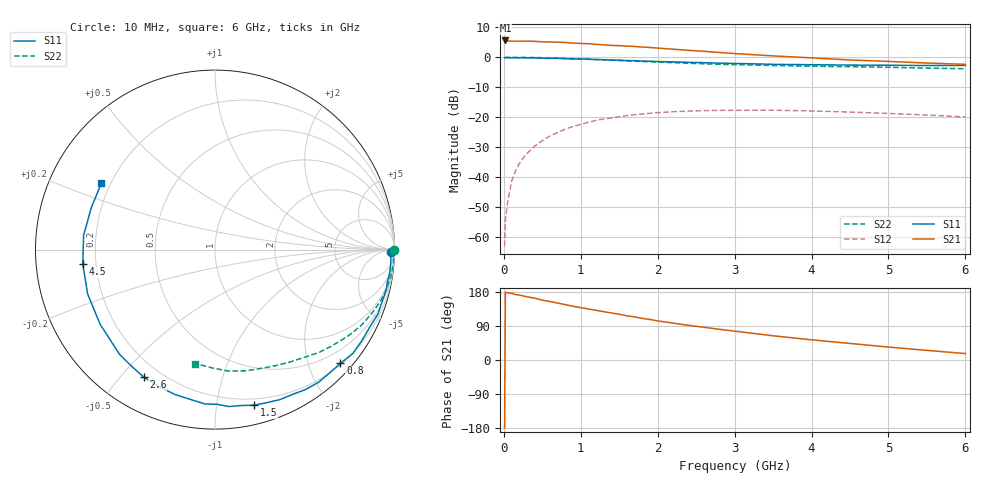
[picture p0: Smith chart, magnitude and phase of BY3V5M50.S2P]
! SIEMENS Small Signal Semiconductors
! BFY420
! Si NPN RF SIEGET Grounded Emitter Transistor in MICRO-X
! VCE = 3.5 V  IC = 0.5 mA
! Common Emitter S-Parameters:  October  1996
# GHz  S  MA  R  50
!  f  S11  S21  S12  S22
! GHz  MAG  ANG  MAG  ANG  MAG  ANG  MAG  ANG
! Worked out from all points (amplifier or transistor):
!   36 points, 10 MHz to 6 GHz, reference 50 ohm
!   highest |S21| = 5.6 dB at 20 MHz (marker M1)
!   |S21| within 3 dB of that: start of sweep to 2.243 GHz
!   unconditionally stable (mu >= 1): 4.7 GHz to end of sweep
!   at 250 MHz: K = 0.04, MSG = 19.5 dB, |S12| = -33.7 dB
!   at 1.4 GHz: K = 0.16, MSG = 12.1 dB, |S12| = -20.3 dB
!   at 6 GHz: K = 1.45, MAG = 4.8 dB, |S12| = -19.9 dB
!   S11 on the Smith chart (normalised r, x): 10 MHz: 76, -51; 800 MHz: 0.22, -2.57; 1.5 GHz: 0.15, -1.27; 2.6 GHz: 0.14, -0.58; 4.5 GHz: 0.15, -0.05; 6 GHz: 0.17, +0.26
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0.01  0.9821 -0.7  1.893 -179.3  0.0007 91.1  0.9999 -0.2
0.02  0.9848 -1.4  1.91 178.7  0.0019 87.8  0.9948 -0.4
0.05  0.9809 -2.7  1.871 177.3  0.0038 87.3  0.999 -1.2
0.1  0.9827 -5.3  1.862 176.1  0.0084 89.3  0.9959 -2.4
0.15  0.9814 -8.1  1.862 172.8  0.0125 82.4  0.9963 -3.6
0.2  0.9764 -10.8  1.857 171.5  0.0167 82.4  0.9976 -4.8
0.3  0.9758 -16.0  1.86 166.7  0.0247 80.7  0.9933 -7.3
0.4  0.9765 -21.5  1.846 163.3  0.0328 77.3  0.9889 -9.6
0.5  0.9643 -26.7  1.812 157.8  0.0406 73.6  0.982 -12.0
0.7  0.9617 -37.0  1.792 150.2  0.0557 67.2  0.968 -16.6
0.8  0.9436 -42.2  1.765 146.0  0.0631 63.6  0.9579 -18.9
1.1  0.9282 -57.2  1.687 134.7  0.0822 54.6  0.9275 -25.3
1.5  0.8941 -75.8  1.564 120.7  0.1018 43.3  0.8833 -33.0
1.8  0.8617 -89.3  1.482 109.7  0.1127 35.9  0.8505 -38.2
2.2  0.8376 -105.4  1.365 97.3  0.1233 26.5  0.8149 -44.8
2.6  0.8136 -119.3  1.258 86.4  0.1281 18.9  0.7788 -50.6
3  0.7896 -132.3  1.154 76.2  0.1302 12.2  0.7534 -56.2
3.5  0.7632 -147.0  1.055 63.9  0.1305 5.1  0.7289 -62.6
4  0.7515 -160.8  0.978 53.3  0.127 -0.5  0.7091 -69.1
4.5  0.741 -173.7  0.902 43.7  0.1216 -5.2  0.6962 -76.0
5.5  0.7279 161.2  0.801 25.4  0.1083 -9.8  0.6594 -91.3
6  0.7331 149.7  0.763 17.0  0.1009 -9.5  0.6442 -99.9
